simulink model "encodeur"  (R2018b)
settings: Solver=VariableStepAuto  StartTime=0.0  StopTime=2  RelTol=1e-3  EnableMultiTasking=on
libraries: simulink x3

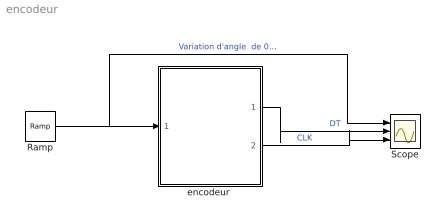
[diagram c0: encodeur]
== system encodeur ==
  Ramp : simulink/Sources/Ramp  slope=36  start=0  InitialOutput=0
  Scope : Scope  NumInputPorts=3
  "encodeur " : Subsystem  mask{p=20}
      mask prompts: p "nombre de pas encodeur"
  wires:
  "encodeur "/1(DT) -> Scope/2  "DT"
  Ramp/1 -> Scope/1, "encodeur "/1(têta degré)  "Variation d'angle  de 0 à 360° en 10s"
  "encodeur "/2(Clk) -> Scope/3  "CLK"

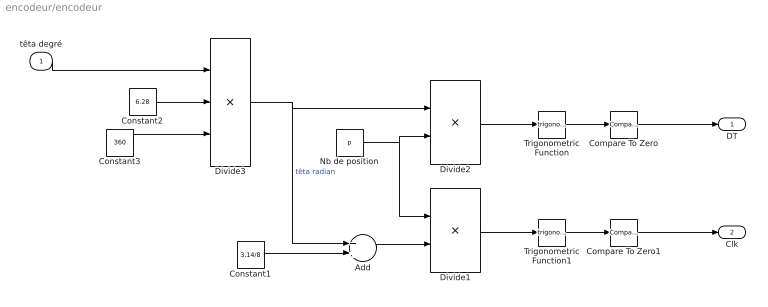
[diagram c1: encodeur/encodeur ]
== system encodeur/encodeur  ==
  têta degré : Inport
  Add : Sum
  Compare To Zero : simulink/Logic and Bit Operations/Compare To Zero  relop=<=  OutDataTypeStr=uint8
  Compare To Zero1 : simulink/Logic and Bit Operations/Compare To Zero  relop=<=  OutDataTypeStr=uint8
  Constant1 : Constant  Value=3.14/8
  Constant2 : Constant  Value=6.28
  Constant3 : Constant  Value=360
  Divide1 : Product  Inputs=**
  Divide2 : Product  Inputs=**
  Divide3 : Product  Inputs=**/
  Nb de position : Constant  Value=p
  Trigonometric Function : Trigonometry
  Trigonometric Function1 : Trigonometry
  DT : Outport
  Clk : Outport  Port=2
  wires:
  Divide3/1 -> Add/1, Divide2/1  "têta radian"
  Trigonometric Function/1 -> Compare To Zero/1
  Constant3/1 -> Divide3/3
  Constant2/1 -> Divide3/2
  Nb de position/1 -> Divide1/1, Divide2/2
  Divide2/1 -> Trigonometric Function/1
  têta degré/1 -> Divide3/1
  Compare To Zero/1 -> DT/1
  Divide1/1 -> Trigonometric Function1/1
  Compare To Zero1/1 -> Clk/1
  Trigonometric Function1/1 -> Compare To Zero1/1
  Add/1 -> Divide1/2
  Constant1/1 -> Add/2
